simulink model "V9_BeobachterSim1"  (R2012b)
settings: Solver=ode4  SolverMode=SingleTasking  StartTime=0.0  StopTime=10.0  FixedStep=0.001  RelTol=1e-3
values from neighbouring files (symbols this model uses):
  A = [-2 1    [V9_1_Beobachterdesign.m]    (also in V9_2_Beobachterdesign.m; V9_3_Beobachterdesign.m)
  B = [1; 1]    [V9_1_Beobachterdesign.m]    (also in V9_2_Beobachterdesign.m = [0; 1]; V9_3_Beobachterdesign.m = [0; 1])
  C = [1 0]    [V9_1_Beobachterdesign.m]    (also in V9_2_Beobachterdesign.m; V9_3_Beobachterdesign.m; LinProb.m = LinProb(A.GetSize()))
  G = place(A',C',poles)    [V9_1_Beobachterdesign.m]    (also in V9_2_Beobachterdesign.m; V2_6_UTFDiskretizierung.m = tf(1,[1 1]))

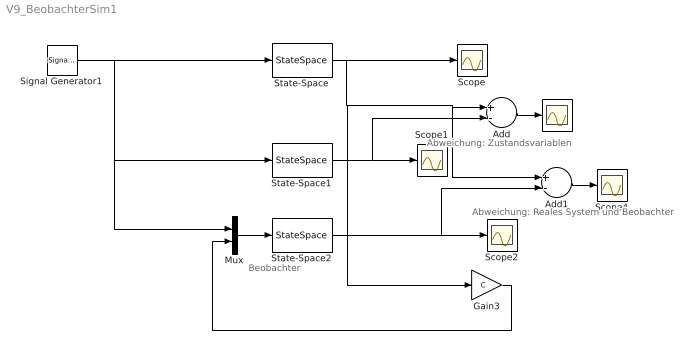
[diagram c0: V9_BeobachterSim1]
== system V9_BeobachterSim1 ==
  note: Abweichung: Zustandsvariablen
  note: Abweichung: Reales System und Beobachter
  note: Beobachter
  " " : Scope
  Add : Sum  Inputs=+-
  Add1 : Sum  Inputs=+-
  Gain3 : Gain  Gain=C  Multiplication=Matrix(K*u)
  Mux : Mux  Inputs=2
  Scope{,1..2,4} (4 alike) : Scope
  Signal Generator1 : SignalGenerator  WaveForm=square  Amplitude=10
  State-Space : StateSpace  A=A  B=B  C=eye(2)  D=[0; 0]  X0=[2; 1]
  State-Space1 : StateSpace  A=A  B=B  C=eye(2)  D=[0; 0]  X0=[0; 0]
  State-Space2 : StateSpace  A=A-G'*C  B=[B G']  C=eye(2)  D=zeros(2,2)  X0=[0; 0]
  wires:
  Mux/1 -> State-Space2/1
  Gain3/1 -> Mux/2
  Signal Generator1/1 -> Mux/1, State-Space1/1, State-Space/1
  State-Space/1 -> Scope/1, Gain3/1, Add1/1, Add/1
  State-Space1/1 -> Scope1/1, Add/2
  Add/1 -> " "/1
  Add1/1 -> Scope4/1
  State-Space2/1 -> Add1/2, Scope2/1
